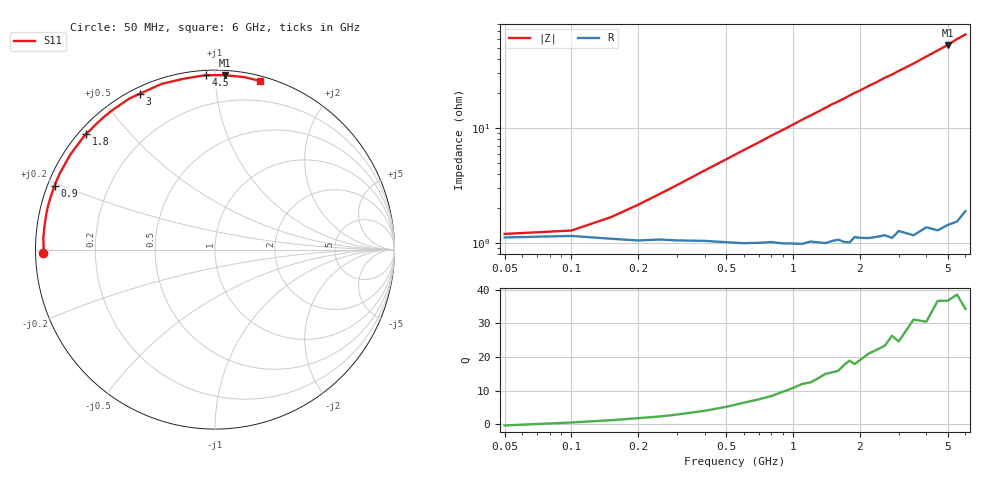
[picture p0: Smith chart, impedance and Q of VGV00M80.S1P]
! Infineon Technologies  Discrete & RF Semiconductors
! BB 831
! Si Tuning Diode in SOD323
! VR =
! S-Parameters:  July  1999
# GHz  S  MA  R  50
!  f  S11
! GHz  MAG  ANG
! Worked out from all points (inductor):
!   34 points, 50 MHz to 6 GHz, reference 50 ohm
!   read as one part to ground: L = 1.68 nH near 400 MHz
!   highest Q = 36.8 at 5 GHz (marker M1), where L = 1.68 nH
!   S11 on the Smith chart (normalised r, x): 50 MHz: 0.02, -0.01; 900 MHz: 0.02, +0.19; 1.8 GHz: 0.02, +0.38; 3 GHz: 0.03, +0.63; 4.5 GHz: 0.03, +0.95; 6 GHz: 0.04, +1.30
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0.05  0.9563 -179.0
0.1  0.9549 178.7
0.15  0.9573 177.1
0.2  0.9588 175.7
0.5  0.9606 168.0
0.7  0.9615 163.1
0.8  0.9612 160.6
0.9  0.9624 158.3
1.1  0.9635 153.5
1.2  0.962 151.2
1.4  0.964 146.7
1.5  0.963 144.4
1.6  0.9624 142.4
1.7  0.9644 140.3
1.8  0.9653 138.1
1.9  0.962 136.0
2  0.963 134.2
2.2  0.9643 130.1
2.4  0.9645 126.5
2.6  0.9646 122.6
2.8  0.9675 119.4
3  0.9641 115.8
3.5  0.9699 107.9
4  0.9683 100.1
4.5  0.9732 93.1
5  0.9732 86.8
5.5  0.9748 80.2
6  0.9723 75.0
